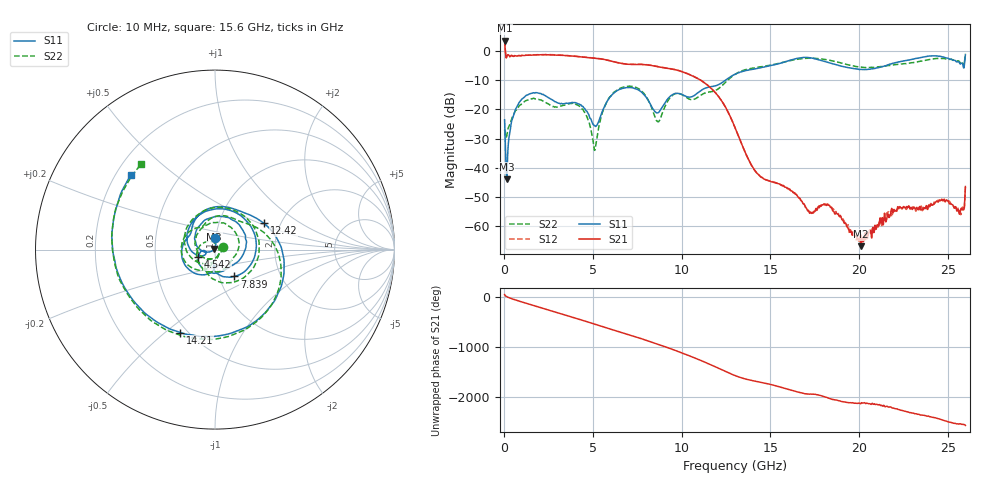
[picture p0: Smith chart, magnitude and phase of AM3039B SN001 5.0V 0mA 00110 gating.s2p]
!Agilent Technologies,E8364B,MY43040894,A.07.50.67
!Agilent E8364B: A.07.50.67
!Date: Tuesday, June 28, 2016 08:04:37
!Correction: S11(Full 2 Port(1,2))
!S21(Full 2 Port(1,2))
!S12(Full 2 Port(1,2))
!S22(Full 2 Port(1,2))
!S2P File: Measurements: S11, S21, S12, S22:
# Hz S  dB  R 50
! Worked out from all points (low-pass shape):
!   1601 points, 10 MHz to 26 GHz, reference 50 ohm
!   highest |S21| = 3.60 dB at 10 MHz (marker M1); lowest = -66.9 dB at 20.12 GHz (marker M2)
!   |S21| within 3 dB of the highest: start of sweep to 44.53 MHz
!   lowest |S11| = -43.9 dB at 123.7 MHz (marker M3), VSWR 1.01, Z = 49.5 + j0.399 ohm
!   |S11| at or under -10 dB: start of sweep to 12.46 GHz
!   |S22| runs from -34.0 to -0.9 dB; largest |S21 - S12| = 0.025
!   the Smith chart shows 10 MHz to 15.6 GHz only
!   S11 on the Smith chart (normalised r, x): 10 MHz: 0.99, +0.13; 4.542 GHz: 0.83, -0.07; 7.839 GHz: 1.18, -0.37; 12.42 GHz: 1.64, +0.53; 14.21 GHz: 0.46, -0.56; 15.6 GHz: 0.26, +0.36
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1e7  -23.53 91.1  3.60 40.6  3.66 41.4  -26.94 17.7
1.237062e8  -43.94 140.7  -2.06 1.4  -2.01 1.5  -29.29 -59.9
7.734562e8  -18.30 155.7  -1.56 -83.5  -1.50 -83.3  -19.33 172.7
1.601888e9  -14.35 70.3  -1.32 -171.8  -1.27 -171.6  -16.25 75.4
2.47905e9  -15.94 -9.6  -1.26 95.7  -1.19 95.8  -18.10 -7.8
3.291238e9  -18.05 -57.8  -1.45 9.2  -1.40 9.3  -18.59 -58.9
4.347081e9  -18.74 -139.4  -2.00 -104.5  -1.96 -104.5  -19.61 -167.6
4.542006e9  -19.75 -155.4  -2.12 -125.6  -2.07 -125.6  -21.13 166.6
5.776531e9  -17.37 -178.7  -3.06 97.5  -3.02 97.6  -17.37 -157.3
6.702425e9  -12.69 76.3  -4.33 -2.6  -4.29 -2.7  -12.37 73.1
7.839488e9  -14.69 -54.4  -4.61 -128.4  -4.56 -128.3  -14.32 -74.4
8.684162e9  -21.07 -90.8  -5.38 130.5  -5.33 130.5  -24.24 -113.1
1.242022e10  -10.18 28.3  -18.68 -37.6  -18.68 -38.4  -10.98 21.4
1.3005e10  -7.94 -16.2  -26.19 -126.9  -26.27 -127.8  -7.95 -23.5
1.420704e10  -6.01 -112.7  -41.66 118.6  -41.56 117.7  -5.60 -123.3
1.5604e10  -4.07 138.3  -45.91 0.7  -45.77 0.5  -4.02 130.8
1.734208e10  -2.38 -21.2  -55.60 -134.9  -55.38 -136.8  -2.44 -14.4
2.011976e10  -6.25 117.0  -66.89 46.2  -63.24 41.1  -5.49 126.4
2.167916e10  -4.58 13.5  -56.94 -33.0  -55.87 -40.9  -4.95 18.5
2.309237e10  -2.70 -92.6  -53.43 -156.4  -54.20 -158.3  -3.89 -83.6
2.419694e10  -1.61 177.9  -52.55 123.1  -52.39 126.0  -2.64 -167.9
2.6e10  -1.29 -24.3  -46.45 -36.3  -46.68 -36.7  -0.88 3.1
